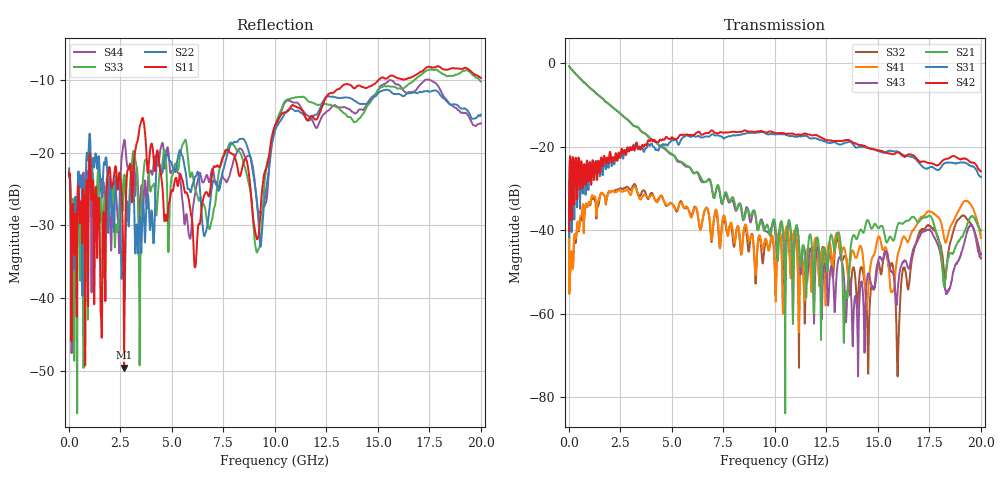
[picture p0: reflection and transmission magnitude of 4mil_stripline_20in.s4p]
! FILE: C:\Archive\Backplane\4-mil striplines\4mil_stripline_20in.s4p
! SMA ->1inch 21mil width microstrip -> 20 inch 4-mil width stripline -> 1 inch 21mil width microstrip -> SMA
! Port 1 -> Port 2, Port 3 -> Port 4
!  1 ----xxxxxxxxxxxxxxxxxx---- 2
!  xxxxxxxxxxxxxxxxxx
!  (Input) xxxxxxxxxxxxxxxxxx  (Output)
!  xxxxxxxxxxxxxxxxxx
!  3 ----xxxxxxxxxxxxxxxxxx---- 4
! 10/8/08
# MHz S DB R 50.00
! FREQ  S11  S12  S13  S14
!  S21  S22  S23  S24
!  S31  S32  S33  S34
!  S41  S42  S43  S44
!  DB  ANG  DB  ANG  DB  ANG  DB  ANG
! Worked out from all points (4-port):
!   2000 points, 10 MHz to 20 GHz, reference 50 ohm
!   strongest paths, dB at 10 MHz, 5.01 GHz, 10.01 GHz, 15.01 GHz, 20 GHz:
!     S42: -40.1, -17.7, -16.7, -20.8, -25.9
!     S31: -41.6, -18.2, -17.0, -21.0, -27.3
!     S21: -0.7, -21.7, -38.3, -39.4, -40.0
!     S43: -0.7, -21.9, -40.2, -47.6, -45.6
!     S41: -33.2, -33.7, -51.4, -41.6, -41.9
!     S32: -31.6, -33.7, -52.1, -47.6, -46.8
!   lowest |S11| = -49.6 dB at 2.68 GHz (marker M1), VSWR 1.01, Z = 50.3 - j0.149 ohm
!   |S11| at or under -10 dB: start of sweep to 15.02 GHz
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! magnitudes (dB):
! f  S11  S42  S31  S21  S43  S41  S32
! 10 MHz  -22.7  -40.1  -41.6  -0.7  -0.7  -33.2  -31.6
! 2.68 GHz  -49.6  -20.9  -21.3  -12.8  -12.9  -30.5  -29.8
! 13.41 GHz  -10.6  -18.4  -19.0  -55.9  -56.9  -45.0  -46.2
! 15.38 GHz  -9.8  -21.4  -21.3  -42.4  -45.1  -44.1  -45.0
! 15.98 GHz  -9.7  -21.3  -21.2  -38.5  -53.3  -45.5  -71.1
! 17.07 GHz  -8.9  -23.6  -24.2  -37.5  -41.1  -37.0  -39.9
! 20 GHz  -9.7  -25.9  -27.3  -40.0  -45.6  -41.9  -46.8
